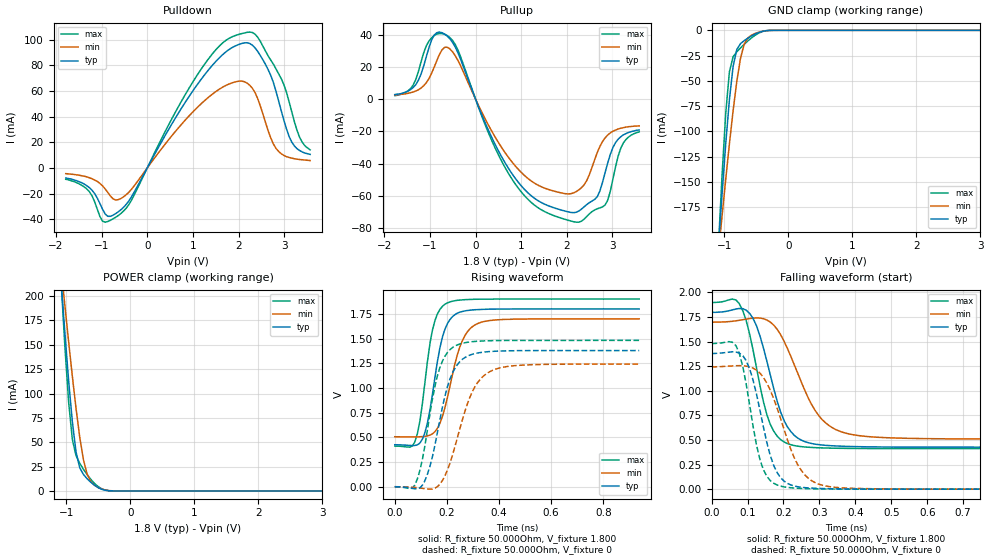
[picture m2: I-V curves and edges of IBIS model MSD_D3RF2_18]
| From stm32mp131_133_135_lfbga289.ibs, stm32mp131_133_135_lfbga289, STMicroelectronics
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[Model] MSD_D3RF2_18
Model_type   I/O
C_comp 2.228pF   2.149pF   2.345pF
Vinh = 1.150V
Vinl = 650.000mV
Vmeas = 900.000mV
Vref = 900.000mV
[Model Spec]
Vinh   1.150V   1.100V   1.200V
Vinl   650.000mV   600.000mV   700.000mV
Vmeas   900.000mV   850.000mV   950.000mV
Vref   900.000mV   850.000mV   950.000mV
[Temperature Range]   25.000   125.000   -40.000
[Voltage Range]   1.800V   1.700V   1.900V
[GND Clamp Reference]   0.00V   0.00V   0.00V
[Pulldown Reference]   0.00V   0.00V   0.00V
[POWER Clamp Reference]   1.800V   1.700V   1.900V
[Pullup Reference]   1.800V   1.700V   1.900V
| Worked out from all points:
|   slope of the pulldown table from 0 to 0.27 V, typ, clamps not added: 15.3 ohm
|   slope of the pullup table from 0 to 0.27 V, typ, clamps not added: 14.6 ohm
|   GND clamp passes 1 mA (typ) near -0.41 V on its own axis
|   POWER clamp passes 1 mA (typ) near -0.41 V on its own axis
|   rising waveform, R_fixture 50.000Ohm, V_fixture 1.800: 20-80 % time 54.8ps typ, 70.2ps min, 47.5ps max; typ from 0.426 V to 1.8 V
|   rising waveform, R_fixture 50.000Ohm, V_fixture 0: 20-80 % time 72ps typ, 90.8ps min, 63.4ps max; typ from 0.001 V to 1.38 V
|   falling waveform, R_fixture 50.000Ohm, V_fixture 1.800: 20-80 % time 64ps typ, 91.1ps min, 54.2ps max; typ from 1.8 V to 0.427 V
|   falling waveform, R_fixture 50.000Ohm, V_fixture 0: 20-80 % time 53.8ps typ, 75.1ps min, 44.8ps max; typ from 1.38 V to 0 V
[GND Clamp]
-1.785V   -901.2mA   -688.7mA   -1.21A
-1.094V   -214.6mA   -220.9mA   -215.3mA
-1.036V   -161.8mA   -183.6mA   -143.3mA
-978.8mV  -112.2mA   -147.3mA   -82mA
-921.2mV  -68.48mA   -112.3mA   -40.93mA
-863.6mV  -35.72mA   -79.61mA   -26.14mA
-806.1mV  -18.98mA   -50.61mA   -21.24mA
-748.5mV  -13.21mA   -27.8mA    -17.43mA
-690.9mV  -10.21mA   -13.79mA   -13.87mA
-575.8mV  -5.519mA   -4.737mA   -7.464mA
-287.9mV  -70.53uA   -119uA     -55.71uA
3.57V     33.94nA    572.8nA    3.717nA
[Power Clamp]
-1.77V    882.6mA    689.8mA    1.159A
-1.079V   212.4mA    226.5mA    212.1mA
-1.021V   160.9mA    189.3mA    146.7mA
-963.6mV  112.9mA    152.9mA    90.89mA
-906.1mV  71.15mA    117.8mA    52.89mA
-848.5mV  40.01mA    84.75mA    36.15mA
-790.9mV  23.77mA    55.41mA    28.47mA
-733.3mV  16.96mA    32.2mA     22.3mA
-618.2mV  8.941mA    9.722mA    11.92mA
-503mV    3.409mA    3.507mA    4.442mA
-272.7mV  29.94uA    100.2uA    29.64uA
3.585V    -51.59nA   -929.3nA   -5.523nA
[Pulldown]
-1.785V   -7.8mA     -4.4mA     -8.8mA
-1.267V   -15.3mA    -7.6mA     -18.5mA
-978.8mV  -32.1mA    -13.9mA    -41.4mA
-575.8mV  -32.49mA   -23.75mA   -35.41mA
1.209V    70.38mA    50.93mA    78.44mA
1.67V     88.85mA    63.32mA    97.95mA
2.188V    97.57mA    66.1mA     105.7mA
2.533V    84.34mA    42.16mA    94.93mA
2.821V    59.8mA     15.3mA     77.19mA
3.167V    20.2mA     7.7mA      43.7mA
3.339V    13.6mA     6.6mA      23.9mA
3.57V     10.6mA     5.8mA      14.1mA
[Pullup]
-1.77V    2.8mA      2.5mA      2.153mA
-1.367V   7.2mA      4.395mA    8.716mA
-1.136V   20.6mA     8.305mA    28.66mA
-906.1mV  39.65mA    19.85mA    39.36mA
-618.2mV  38.98mA    32.14mA    39.33mA
878.8mV   -49.38mA   -41.65mA   -52.89mA
1.455V    -64.25mA   -54.44mA   -68.75mA
2.203V    -70.07mA   -57.29mA   -76.21mA
2.664V    -60.51mA   -33.26mA   -67.93mA
2.836V    -45.7mA    -24.05mA   -65.6mA
3.182V    -23.3mA    -18.01mA   -30.35mA
3.585V    -19.1mA    -16.55mA   -20.27mA
[Ramp]
R_load=50.000Ohm
dV/dt_r   825.630mV/64.500ps  729.899mV/81.500ps  890.610mV/56.000ps
dV/dt_f   825.630mV/60.000ps  729.899mV/84.000ps  890.610mV/50.000ps
[Rising waveform]
R_fixture=50.000Ohm
V_fixture=1.800
V_fixture_min=1.700
V_fixture_max=1.900
0s        426.1mV    506.8mV    412.6mV
68ps      417.8mV    505.1mV    415mV
87ps      425mV      505.7mV    540mV
106ps     482.3mV    508.3mV    842.7mV
144ps     925.9mV    534.8mV    1.579V
173ps     1.403V     640.9mV    1.794V
192ps     1.591V     795.8mV    1.847V
250ps     1.768V     1.418V     1.89V
317ps     1.793V     1.651V     1.898V
938ps     1.8V       1.7V       1.9V
[Rising waveform]
R_fixture=50.000Ohm
V_fixture=0
0s        1.121mV    1mV        1.034mV
77ps      -19.82mV   -6.525mV   17.45mV
115ps     59mV       -18.36mV   406.7mV
144ps     299mV      -22.33mV   880mV
173ps     677.2mV    26.5mV     1.206V
202ps     1.012V     169mV      1.359V
230ps     1.195V     398.9mV    1.424V
298ps     1.342V     965.2mV    1.469V
374ps     1.37V      1.177V     1.479V
938ps     1.379V     1.242V     1.482V
[Falling waveform]
R_fixture=50.000Ohm
V_fixture=1.800
V_fixture_min=1.700
V_fixture_max=1.900
0s        1.798V     1.698V     1.898V
77ps      1.837V     1.717V     1.887V
96ps      1.821V     1.729V     1.719V
115ps     1.739V     1.739V     1.422V
144ps     1.44V      1.734V     893.4mV
163ps     1.167V     1.7V       662.4mV
211ps     633.7mV    1.431V     463.5mV
288ps     457.7mV    800.8mV    422.5mV
365ps     436.5mV    578.5mV    415.2mV
938ps     427.1mV    509.5mV    412.8mV
[Falling waveform]
R_fixture=50.000Ohm
V_fixture=0
0s        1.379V     1.243V     1.481V
68ps      1.394V     1.255V     1.459V
96ps      1.308V     1.251V     1.075V
115ps     1.115V     1.232V     649.8mV
135ps     796.4mV    1.178V     296.1mV
163ps     346.1mV    1.009V     88.39mV
183ps     164.8mV    817mV      41.65mV
240ps     24.42mV    246.4mV    9.192mV
307ps     6.557mV    41.18mV    2.243mV
938ps     3.551uV    18uV       1.049uV
